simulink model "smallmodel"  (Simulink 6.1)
settings: Solver=ode5  StartTime=0.0  StopTime=300.0  FixedStep=0.001  RelTol=1e-3

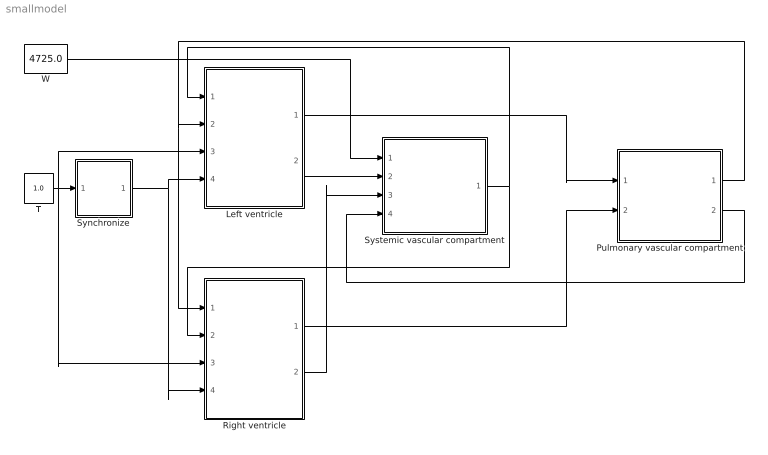
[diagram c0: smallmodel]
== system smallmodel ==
  Left ventricle : Subsystem
  Pulmonary vascular compartment : Subsystem
  Right ventricle : Subsystem
  Synchronize : Subsystem
  Systemic vascular compartment : Subsystem
  T : Constant  Value=1.0
  W : Constant  Value=4725.0
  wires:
  Pulmonary vascular compartment/2(VPR) -> Systemic vascular compartment/4(VPR)
  T/1 -> Left ventricle/3(T), Synchronize/1(T), Right ventricle/3(T)
  Synchronize/1(CT) -> Left ventricle/4(CT), Right ventricle/4(CT)
  Left ventricle/2(VHL) -> Systemic vascular compartment/2(VHL)
  Left ventricle/1(FPRHL) -> Pulmonary vascular compartment/1(FPRHL)
  Systemic vascular compartment/1(PPL) -> Left ventricle/1(PPL), Right ventricle/2(PPL)
  Pulmonary vascular compartment/1(PPR) -> Left ventricle/2(PPR), Right ventricle/1(PPR)
  Right ventricle/2(VHR) -> Systemic vascular compartment/3(VHR)
  Right ventricle/1(FHRPR) -> Pulmonary vascular compartment/2(FHRPR)
  W/1 -> Systemic vascular compartment/1(W)

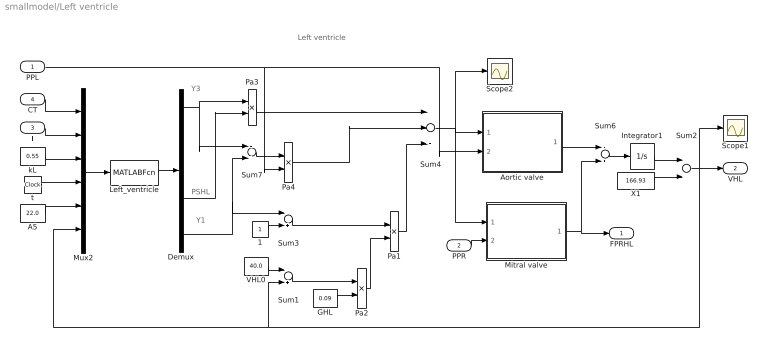
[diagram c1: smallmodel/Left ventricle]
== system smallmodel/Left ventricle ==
  note: Left ventricle
  note: Y1
  note: Y3
  note: PSHL
  PPL : Inport  Port=1  LatchInput=off
  PPR : Inport  Port=2  LatchInput=off
  T : Inport  Port=3  LatchInput=off
  CT : Inport  Port=4  LatchInput=off
  1 : Constant
  A5 : Constant  Value=22.0
  Aortic valve : Subsystem
  Demux : Demux  Outputs=8
  GHL : Constant  Value=0.09
  Integrator1 : Integrator
  Left_ventricle : MATLABFcn  MATLABFcn=left_ventricle  OutputDimensions=8
  Mitral valve : Subsystem
  Mux2 : Mux  Inputs=6
  Pa{1..4} (4 alike) : Product  Inputs=**
  Scope1 : Scope
  Scope2 : Scope
  Sum{1,3,6..7} (4 alike) : Sum  Inputs=-+
  Sum2 : Sum
  Sum4 : Sum  Inputs=+++
  VHL0 : Constant  Value=40.0
  X1 : Constant  Value=166.93
  kL : Constant  Value=0.55
  t : Clock
  FPRHL : Outport
  VHL : Outport  Port=2
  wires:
  Mux2/1 -> Left_ventricle/1
  Left_ventricle/1 -> Demux/1
  CT/1 -> Mux2/1
  T/1 -> Mux2/2
  kL/1 -> Mux2/3
  t/1 -> Mux2/4
  A5/1 -> Mux2/5
  Demux/8 -> Sum7/2, Sum3/1
  Demux/1 -> Pa3/1, Sum7/1
  Demux/6 -> Pa3/2
  1/1 -> Sum3/2
  VHL0/1 -> Sum1/1
  Sum1/1 -> Pa2/1
  GHL/1 -> Pa2/2
  Pa2/1 -> Pa1/2
  Sum3/1 -> Pa1/1
  Pa1/1 -> Sum4/3
  Sum7/1 -> Pa4/1
  Pa4/1 -> Sum4/2
  Pa3/1 -> Sum4/1
  PPL/1 -> Pa4/2, Aortic valve/2(PPL)
  Sum4/1 -> Aortic valve/1(PHL), Scope2/1, Mitral valve/1(PHL)
  PPR/1 -> Mitral valve/2(PPR)
  Aortic valve/1(FHLPL) -> Sum6/1
  Mitral valve/1(FPRHL) -> Sum6/2, FPRHL/1
  Sum6/1 -> Integrator1/1
  Integrator1/1 -> Sum2/1
  X1/1 -> Sum2/2
  Sum2/1 -> VHL/1, Scope1/1, Mux2/6, Sum1/2

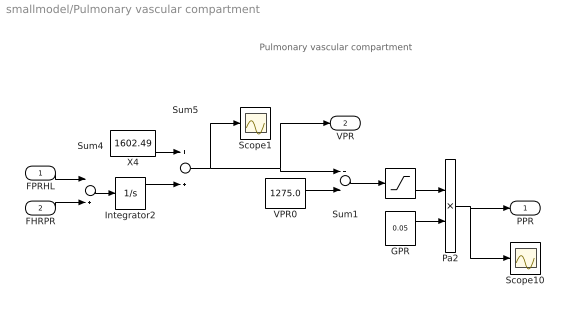
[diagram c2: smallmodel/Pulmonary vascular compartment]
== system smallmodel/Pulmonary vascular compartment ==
  note: Pulmonary vascular compartment
  FPRHL : Inport  Port=1  LatchInput=off
  FHRPR : Inport  Port=2  LatchInput=off
  " " : Saturate  UpperLimit=1000  LowerLimit=0
  GPR : Constant  Value=0.05
  Integrator2 : Integrator
  Pa2 : Product  Inputs=**
  Scope1 : Scope
  Scope10 : Scope
  Sum1 : Sum  Inputs=+-
  Sum4 : Sum  Inputs=-+
  Sum5 : Sum
  VPR0 : Constant  Value=1275.0
  X4 : Constant  Value=1602.49
  PPR : Outport
  VPR : Outport  Port=2
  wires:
  VPR0/1 -> Sum1/2
  Sum4/1 -> Integrator2/1
  X4/1 -> Sum5/1
  FHRPR/1 -> Sum4/2
  FPRHL/1 -> Sum4/1
  Sum5/1 -> VPR/1, Sum1/1, Scope1/1
  Integrator2/1 -> Sum5/2
  Sum1/1 -> " "/1
  " "/1 -> Pa2/1
  Pa2/1 -> PPR/1, Scope10/1
  GPR/1 -> Pa2/2

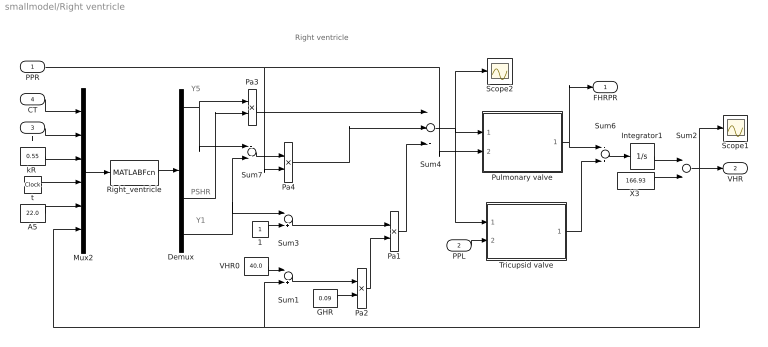
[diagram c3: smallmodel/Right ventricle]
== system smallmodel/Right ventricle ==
  note: Right ventricle
  note: Y1
  note: Y5
  note: PSHR
  PPR : Inport  Port=1  LatchInput=off
  PPL : Inport  Port=2  LatchInput=off
  T : Inport  Port=3  LatchInput=off
  CT : Inport  Port=4  LatchInput=off
  1 : Constant
  A5 : Constant  Value=22.0
  Demux : Demux  Outputs=8
  GHR : Constant  Value=0.09
  Integrator1 : Integrator
  Mux2 : Mux  Inputs=6
  Pa{1..4} (4 alike) : Product  Inputs=**
  Pulmonary valve : Subsystem
  Right_ventricle : MATLABFcn  MATLABFcn=right_ventricle  OutputDimensions=8
  Scope1 : Scope
  Scope2 : Scope
  Sum{1,3,6..7} (4 alike) : Sum  Inputs=-+
  Sum2 : Sum
  Sum4 : Sum  Inputs=+++
  Tricupsid valve : Subsystem
  VHR0 : Constant  Value=40.0
  "X3 " : Constant  Value=166.93
  "kR " : Constant  Value=0.55
  t : Clock
  FHRPR : Outport
  VHR : Outport  Port=2
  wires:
  Mux2/1 -> Right_ventricle/1
  Right_ventricle/1 -> Demux/1
  CT/1 -> Mux2/1
  T/1 -> Mux2/2
  "kR "/1 -> Mux2/3
  t/1 -> Mux2/4
  A5/1 -> Mux2/5
  Demux/8 -> Sum7/2, Sum3/1
  Demux/1 -> Pa3/1, Sum7/1
  Demux/6 -> Pa3/2
  1/1 -> Sum3/2
  VHR0/1 -> Sum1/1
  Sum1/1 -> Pa2/1
  GHR/1 -> Pa2/2
  Pa2/1 -> Pa1/2
  Sum3/1 -> Pa1/1
  Pa1/1 -> Sum4/3
  Sum7/1 -> Pa4/1
  Pa4/1 -> Sum4/2
  Pa3/1 -> Sum4/1
  PPR/1 -> Pa4/2, Pulmonary valve/2(PPR)
  Sum4/1 -> Pulmonary valve/1(PHR), Scope2/1, Tricupsid valve/1(PHR)
  PPL/1 -> Tricupsid valve/2(PPL)
  Pulmonary valve/1(FHRPR) -> Sum6/1, FHRPR/1
  Tricupsid valve/1(FPLHR) -> Sum6/2
  Sum6/1 -> Integrator1/1
  Integrator1/1 -> Sum2/1
  "X3 "/1 -> Sum2/2
  Sum2/1 -> VHR/1, Scope1/1, Mux2/6, Sum1/2

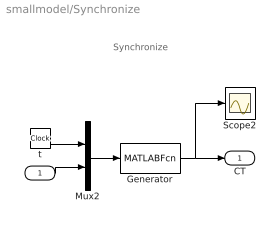
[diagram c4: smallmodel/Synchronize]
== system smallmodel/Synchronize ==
  note: Synchronize
  T : Inport  Port=1  LatchInput=off
  Generator : MATLABFcn  MATLABFcn=time_generator  OutputDimensions=1
  Mux2 : Mux  Inputs=2
  Scope2 : Scope
  t : Clock
  CT : Outport
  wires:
  T/1 -> Mux2/2
  t/1 -> Mux2/1
  Mux2/1 -> Generator/1
  Generator/1 -> Scope2/1, CT/1

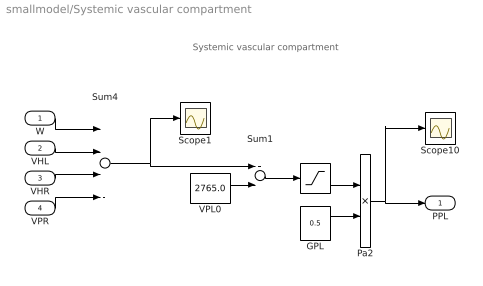
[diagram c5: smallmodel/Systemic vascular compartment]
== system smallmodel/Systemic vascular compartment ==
  note: Systemic vascular compartment
  W : Inport  Port=1  LatchInput=off
  VHL : Inport  Port=2  LatchInput=off
  VHR : Inport  Port=3  LatchInput=off
  VPR : Inport  Port=4  LatchInput=off
  " " : Saturate  UpperLimit=1000  LowerLimit=0
  GPL : Constant  Value=0.5
  Pa2 : Product  Inputs=**
  Scope1 : Scope
  Scope10 : Scope
  Sum1 : Sum  Inputs=+-
  Sum4 : Sum  Inputs=+---
  VPL0 : Constant  Value=2765.0
  PPL : Outport
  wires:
  VPL0/1 -> Sum1/2
  Sum4/1 -> Scope1/1, Sum1/1
  Sum1/1 -> " "/1
  " "/1 -> Pa2/1
  Pa2/1 -> PPL/1, Scope10/1
  GPL/1 -> Pa2/2
  W/1 -> Sum4/1
  VHL/1 -> Sum4/2
  VHR/1 -> Sum4/3
  VPR/1 -> Sum4/4

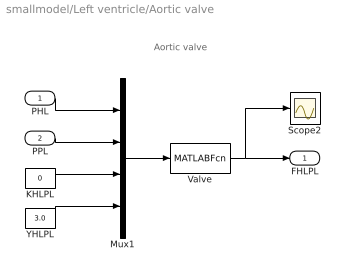
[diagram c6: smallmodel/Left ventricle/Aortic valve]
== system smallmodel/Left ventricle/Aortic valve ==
  note: Aortic valve
  PHL : Inport  Port=1  LatchInput=off
  PPL : Inport  Port=2  LatchInput=off
  KHLPL : Constant  Value=0
  Mux1 : Mux
  Scope2 : Scope
  Valve : MATLABFcn  MATLABFcn=valve  OutputDimensions=1
  YHLPL : Constant  Value=3.0
  FHLPL : Outport
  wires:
  PHL/1 -> Mux1/1
  PPL/1 -> Mux1/2
  KHLPL/1 -> Mux1/3
  Mux1/1 -> Valve/1
  Valve/1 -> FHLPL/1, Scope2/1
  YHLPL/1 -> Mux1/4

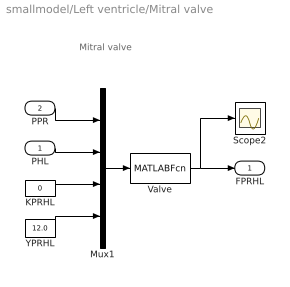
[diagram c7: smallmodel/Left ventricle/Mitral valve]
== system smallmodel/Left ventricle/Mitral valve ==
  note: Mitral valve
  PHL : Inport  Port=1  LatchInput=off
  PPR : Inport  Port=2  LatchInput=off
  KPRHL : Constant  Value=0
  Mux1 : Mux
  Scope2 : Scope
  Valve : MATLABFcn  MATLABFcn=valve  OutputDimensions=1
  YPRHL : Constant  Value=12.0
  FPRHL : Outport
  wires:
  PPR/1 -> Mux1/1
  KPRHL/1 -> Mux1/3
  Mux1/1 -> Valve/1
  Valve/1 -> Scope2/1, FPRHL/1
  PHL/1 -> Mux1/2
  YPRHL/1 -> Mux1/4

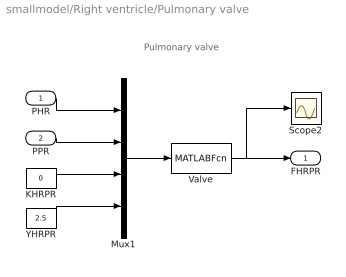
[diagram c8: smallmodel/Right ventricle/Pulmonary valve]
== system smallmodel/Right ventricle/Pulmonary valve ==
  note: Pulmonary valve
  PHR : Inport  Port=1  LatchInput=off
  PPR : Inport  Port=2  LatchInput=off
  KHRPR : Constant  Value=0
  Mux1 : Mux
  Scope2 : Scope
  Valve : MATLABFcn  MATLABFcn=valve  OutputDimensions=1
  YHRPR : Constant  Value=2.5
  FHRPR : Outport
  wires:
  PHR/1 -> Mux1/1
  PPR/1 -> Mux1/2
  KHRPR/1 -> Mux1/3
  Mux1/1 -> Valve/1
  Valve/1 -> FHRPR/1, Scope2/1
  YHRPR/1 -> Mux1/4

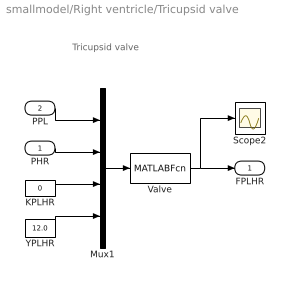
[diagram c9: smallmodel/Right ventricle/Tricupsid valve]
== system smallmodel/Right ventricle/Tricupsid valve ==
  note: Tricupsid valve
  PHR : Inport  Port=1  LatchInput=off
  PPL : Inport  Port=2  LatchInput=off
  KPLHR : Constant  Value=0
  Mux1 : Mux
  Scope2 : Scope
  Valve : MATLABFcn  MATLABFcn=valve  OutputDimensions=1
  YPLHR : Constant  Value=12.0
  FPLHR : Outport
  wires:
  PPL/1 -> Mux1/1
  KPLHR/1 -> Mux1/3
  Mux1/1 -> Valve/1
  Valve/1 -> Scope2/1, FPLHR/1
  PHR/1 -> Mux1/2
  YPLHR/1 -> Mux1/4
